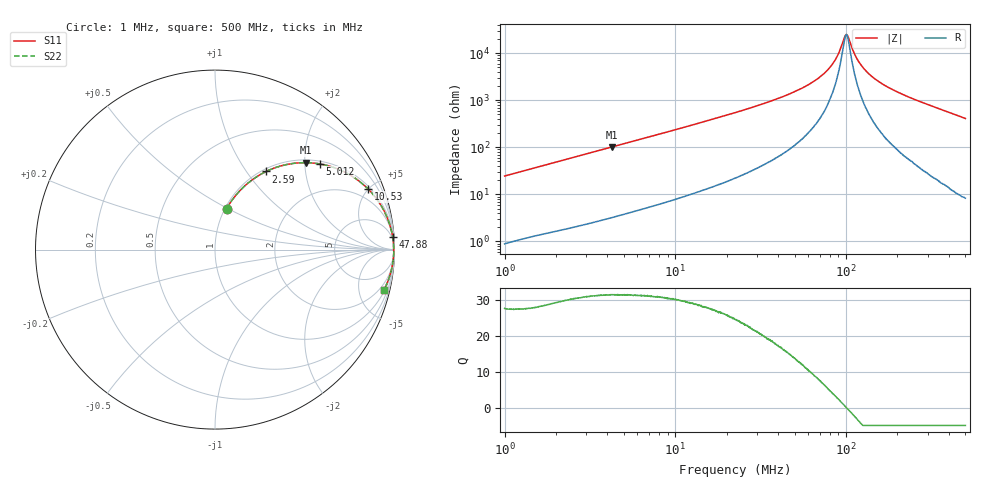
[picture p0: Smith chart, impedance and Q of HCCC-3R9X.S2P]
!s-Parameter Generated by FASTRON Sdn. Bhd.
!FASTRON P/N : HCCC-3R9X
!Keysight Technologies,E4991B,MY54100416,A.01.15
!Date: Thu Apr 02 15:10:34 2026
!Version  : Rev00 Thu Apr 02 15:10:34 2026
!Data & Calibration Information:
!PortZ  Port1:50+j0  Port2:50+j0
!When reading, reference impedance value at option line is always used.
! Remarks : This data is being provided solely for informational purposes.
!Freq	S11	S21	S12	S22
# Hz S dB R 50
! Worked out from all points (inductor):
!   1601 points, 1 MHz to 500 MHz, reference 50 ohm
!   read as one part in series: L = 3.88 uH near 1.032 MHz
!   highest Q = 31.5 at 4.258 MHz (marker M1), where L = 3.79 uH
!   self-resonance near 100.1 MHz
!   S11 on the Smith chart (normalised r, x): 1 MHz: 1.02, +0.49; 2.59 MHz: 1.04, +1.24; 5.012 MHz: 1.08, +2.38; 10.53 MHz: 1.17, +4.98; 47.88 MHz: 3, +28; 500 MHz: 1.17, -8.21
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1000000  -12.53 74.3  -0.33 -13.7  -0.33 -13.7  -12.53 74.3
2589881  -5.68 56.8  -1.54 -31.3  -1.54 -31.3  -5.68 56.8
2820919  -5.17 54.7  -1.76 -33.5  -1.76 -33.5  -5.17 54.7
4257919  -3.09 43.7  -3.21 -44.5  -3.21 -44.5  -3.09 43.7
5012396  -2.45 39.3  -3.97 -48.9  -3.97 -48.9  -2.45 39.3
7957584  -1.19 27.6  -6.69 -60.6  -6.69 -60.6  -1.19 27.6
1.052531e7  -0.75 21.6  -8.68 -66.5  -8.68 -66.5  -0.75 21.6
2.236068e7  -0.21 10.3  -14.93 -77.4  -14.93 -77.4  -0.21 10.3
4.7875e7  -0.06 4.0  -23.10 -82.1  -23.10 -82.1  -0.06 4.0
6.307767e7  -0.05 2.4  -27.52 -81.6  -27.52 -81.6  -0.05 2.4
7.368004e7  -0.04 1.6  -31.13 -79.7  -31.13 -79.7  -0.04 1.6
8.246482e7  -0.04 1.0  -35.00 -75.6  -35.00 -75.6  -0.04 1.0
8.878078e7  -0.04 0.6  -38.75 -68.5  -38.75 -68.5  -0.04 0.6
9.745486e7  -0.04 0.2  -46.33 -33.2  -46.33 -33.2  -0.04 0.2
1.005306e8  -0.03 -0.0  -47.98 0.6  -47.98 0.6  -0.03 -0.0
1.033014e8  -0.03 -0.1  -46.65 31.3  -46.65 31.3  -0.03 -0.1
1.147233e8  -0.03 -0.7  -38.25 70.8  -38.25 70.8  -0.03 -0.7
1.25932e8  -0.04 -1.1  -33.82 78.0  -33.82 78.0  -0.04 -1.1
1.453951e8  -0.04 -1.9  -29.47 81.6  -29.47 81.6  -0.04 -1.9
1.77937e8  -0.05 -3.1  -25.41 82.8  -25.41 82.8  -0.05 -3.1
2.583476e8  -0.08 -5.7  -20.10 82.0  -20.10 82.0  -0.08 -5.7
5e8  -0.29 -13.6  -12.56 75.2  -12.56 75.2  -0.29 -13.6
